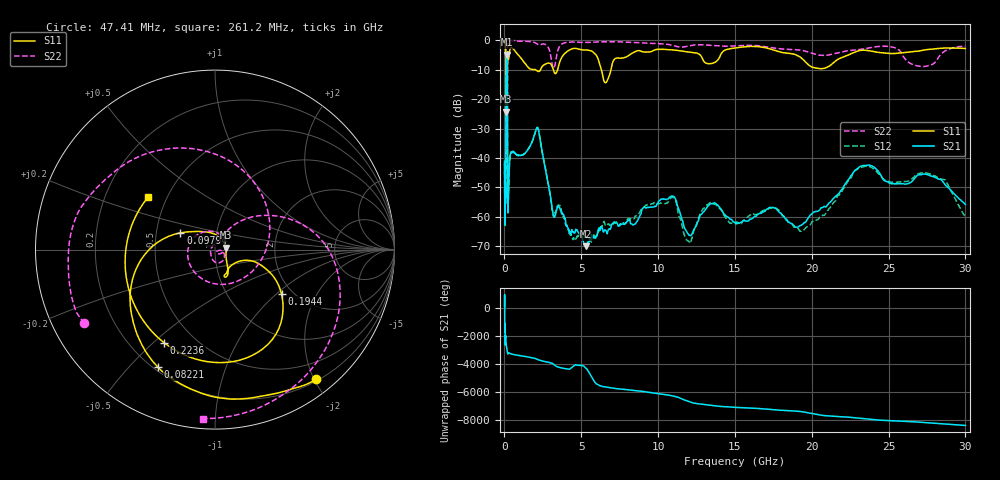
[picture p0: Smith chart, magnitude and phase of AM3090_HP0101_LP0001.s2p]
! Date/Time: Thu, Feb 28, 2019 1:58 PM
! Network Analyzer: Agilent Technologies E8364B Rev: A.07.50.67
! Sweep from 0.010 to 30.000 GHz, 1601 Points, Sweep Type: LOG
! Power Supply: 5.023 V, 0.002 A
# Hz S DB R 50
!freq MagS11 AngS11 MagS21 AngS21 MagS12 AngS12 MagS22 AngS22
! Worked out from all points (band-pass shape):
!   1601 points, 10 MHz to 30 GHz, reference 50 ohm
!   highest |S21| = -4.97 dB at 139.7 MHz (marker M1); lowest = -69.9 dB at 5.285 GHz (marker M2)
!   |S21| within 3 dB of the highest: 106 MHz to 178.4 MHz (72.42 MHz wide, 50.9 % of centre)
!   lowest |S11| = -24.3 dB at 105.1 MHz (marker M3), VSWR 1.13, Z = 56.3 + j1.26 ohm
!   |S11| at or under -10 dB: 1.998 GHz to 2.353 GHz (354.4 MHz wide, 16.3 % of centre); 3.182 GHz to 3.46 GHz (278.9 MHz wide, 8.4 % of centre); 6.307 GHz to 6.932 GHz (625 MHz wide, 9.44 % of centre)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
!   |S22| runs from -36.6 to -0.1 dB; largest |S21 - S12| = 0.013
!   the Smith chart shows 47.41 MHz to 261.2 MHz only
!   S11 on the Smith chart (normalised r, x): 47.41 MHz: 0.23, -2.02; 82.21 MHz: 0.22, -0.61; 97.94 MHz: 0.67, +0.13; 194.4 MHz: 1.75, -1.08; 223.6 MHz: 0.34, -0.54; 261.2 MHz: 0.39, +0.30
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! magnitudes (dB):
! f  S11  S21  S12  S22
! 10 MHz  -0.2  -41.0  -44.7  -0.5
! 38.04 MHz  -0.5  -61.5  -59.4  -1.3
! 47.41 MHz  -0.8  -50.4  -51.8  -1.6
! 82.21 MHz  -2.8  -47.3  -45.0  -5.8
! 97.94 MHz  -13.4  -14.5  -14.5  -15.1
! 105.1 MHz  -24.3  -8.4  -8.4  -17.8
! 139.7 MHz  -16.6  -5.0  -4.9  -31.7
! 144.7 MHz  -16.7  -5.0  -5.0  -25.1
! 171.5 MHz  -16.3  -6.6  -6.6  -33.1
! 194.4 MHz  -7.0  -20.6  -20.5  -8.9
! 223.6 MHz  -4.6  -58.6  -56.4  -1.3
! 261.2 MHz  -6.5  -52.6  -52.8  -0.5
! 550.5 MHz  -3.0  -38.1  -37.7  -0.2
! 2.084 GHz  -10.3  -30.0  -30.0  -1.2
! 3.156 GHz  -9.6  -58.7  -59.3  -9.3
! 5.285 GHz  -3.4  -69.9  -66.9  -0.8
! 6.619 GHz  -14.4  -64.7  -62.4  -0.6
! 7.926 GHz  -5.7  -62.0  -61.5  -0.7
! 10.65 GHz  -3.3  -53.9  -54.9  -1.5
! 19.51 GHz  -7.0  -62.0  -64.3  -3.7
! 23.48 GHz  -3.5  -42.5  -42.8  -2.9
! 30 GHz  -2.9  -55.7  -60.1  -2.1
